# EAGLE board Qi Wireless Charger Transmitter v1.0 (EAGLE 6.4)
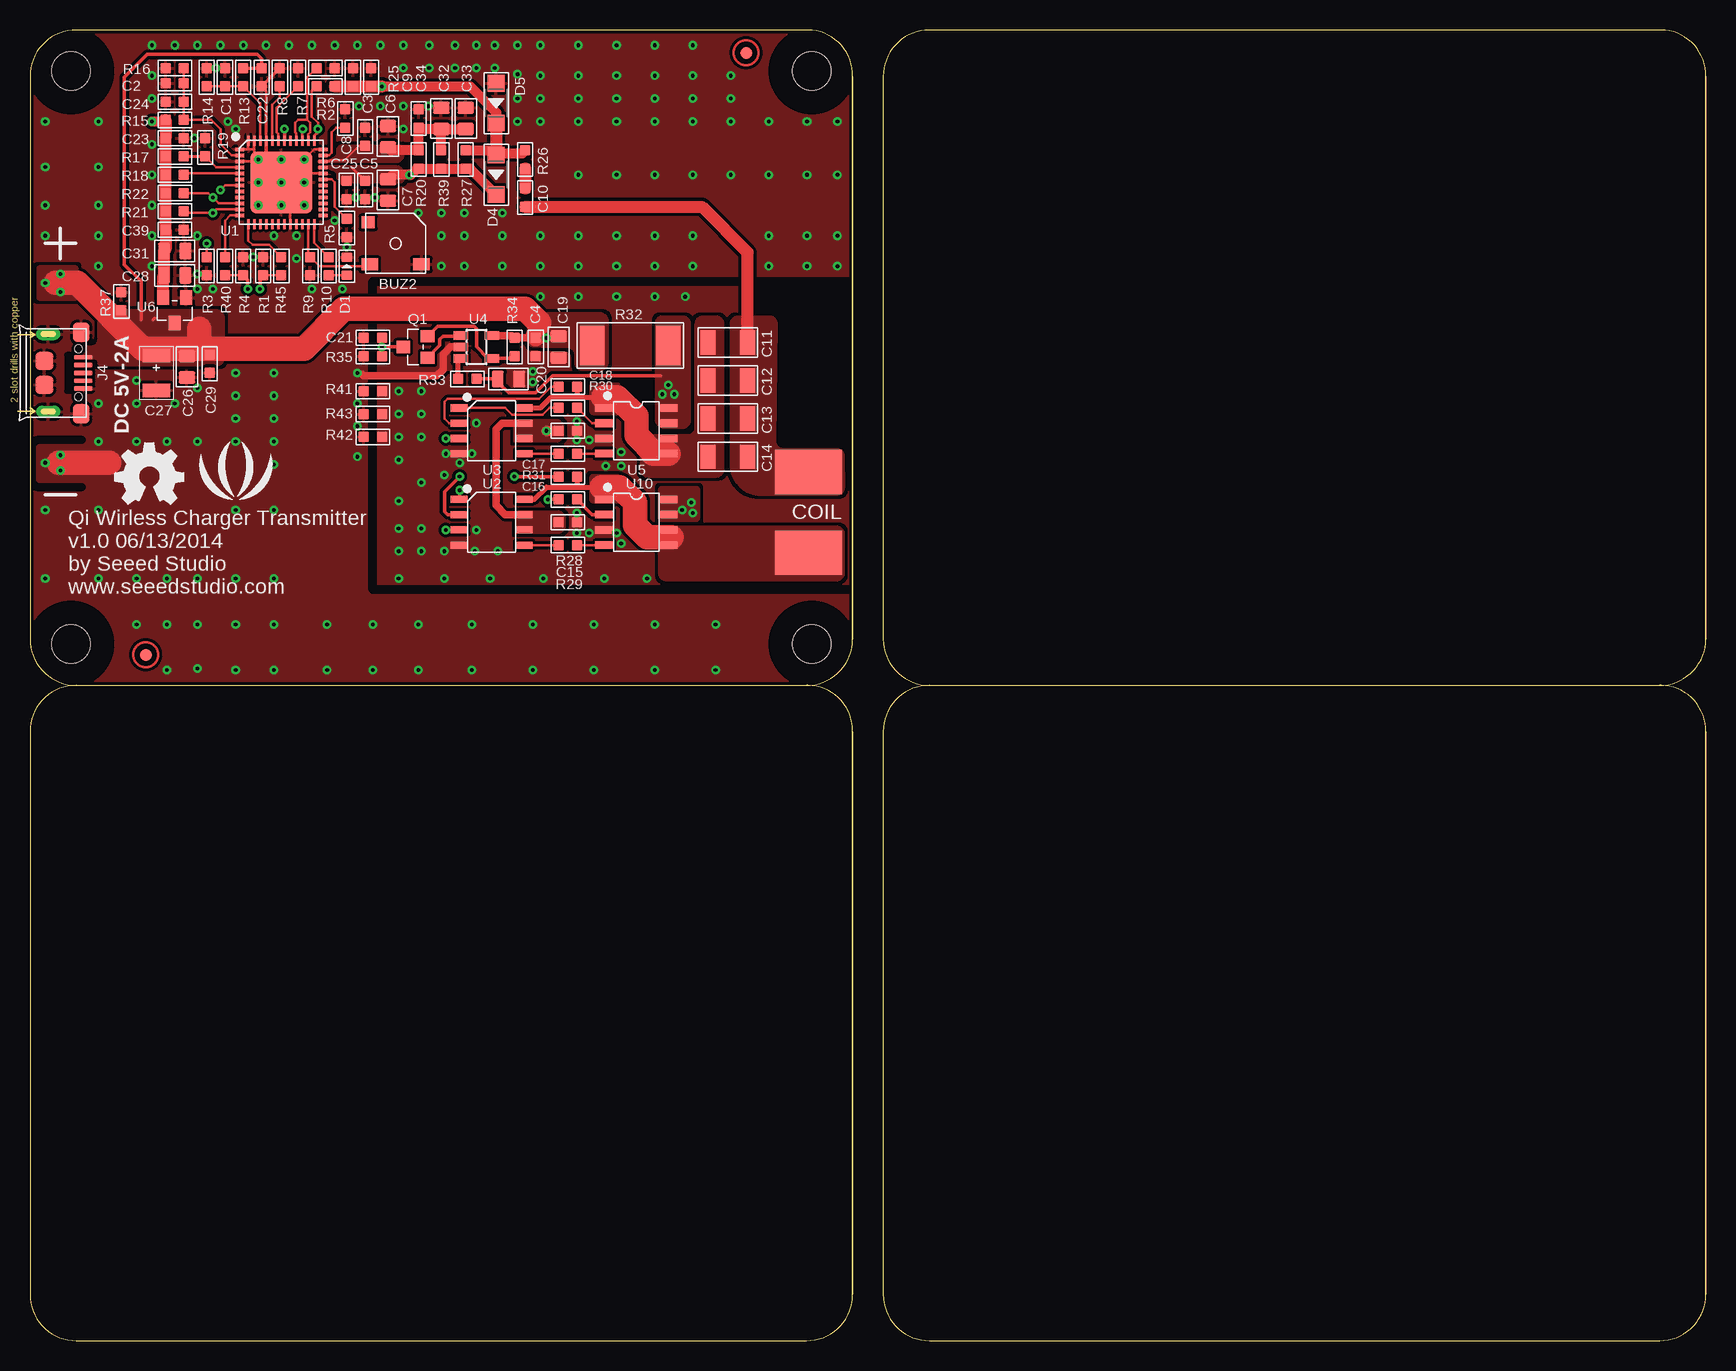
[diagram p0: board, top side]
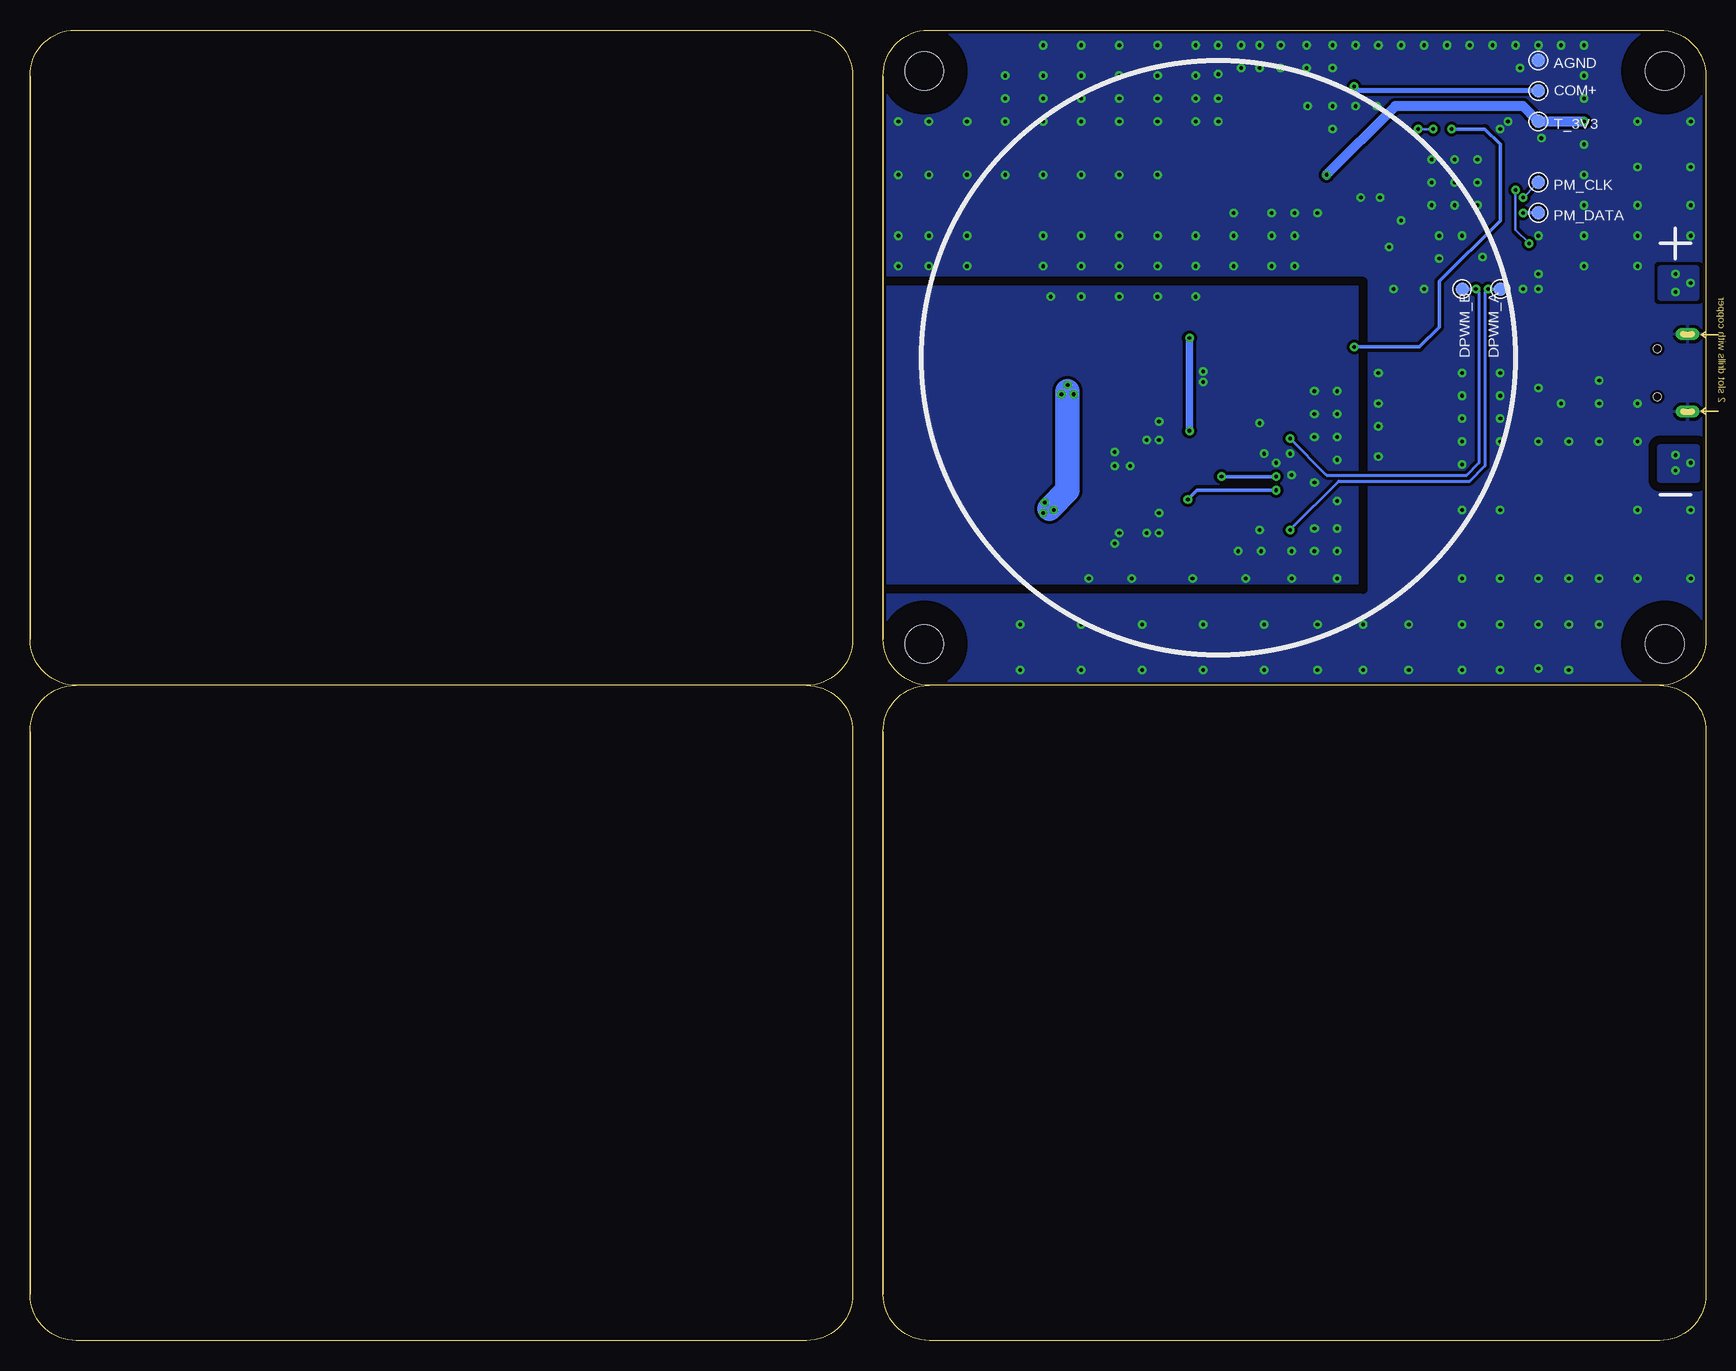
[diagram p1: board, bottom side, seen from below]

Size 139.7 x 109.22 mm. Coordinates in mm from the lower left corner, seen from the top.
Outline: 3.86,54.61 arc-90 0,58.47 0,105.36 arc-90 3.86,109.22 64.85,109.22 arc-90 68.58,105.36 68.58,58.47 arc-90 64.72,54.61
Outline: 3.86,54.61 64.72,54.61
Outline: 64.72,54.61 64.85,54.61 arc-90 68.58,50.75 68.58,3.86 arc-90 64.72,0 3.86,0 arc-90 0,3.86 0,50.75 arc-90 3.86,54.61
Outline: 68.58,50.75 68.58,3.86
Outline: 68.58,105.36 68.58,58.47
Outline: 74.98,54.61 arc-90 71.12,58.47 71.12,105.36 arc-90 74.98,109.22 135.97,109.22 arc-90 139.7,105.36 139.7,58.47 arc-90 135.84,54.61
Outline: 74.98,54.61 135.84,54.61
Outline: 135.84,54.61 135.97,54.61 arc-90 139.7,50.75 139.7,3.86 arc-90 135.84,0 74.98,0 arc-90 71.12,3.86 71.12,50.75 arc-90 74.98,54.61
Outline: 139.7,50.75 139.7,3.86
Outline: 139.7,105.36 139.7,58.47
Copper layers (1*16): Top 0.035mm / dielectric 1.5mm / Bottom 0.035mm
Design rules "default *": minimum track width 8mil, minimum drill 12mil, track to track 6mil, track to pad 6mil, pad to pad 6mil, via to via 6mil, smd to smd 0mil, copper to edge 10mil, drill to drill 8mil, minimum pad ring 10mil, minimum via ring 8mil, stop-mask expansion 4mil, vias tented up to drill 25mil, thermal gap 10mil
Net classes: 0 default: width 0.003 mm, drill 0.254 mm, clearance 0.152 mm
Holes 3.2 mm at 3.43,105.79 3.43,58.04 65.15,58.04 65.15,105.79
Holes 2.03 mm at 7.62,113.66 132.08,113.66 132.08,-4.45 7.62,-4.45
tRestrict: area 0.2,102.5 to 6.7,109; area 0.2,54.8 to 6.7,61.3; area 61.9,54.8 to 68.4,61.3; area 61.9,102.5 to 68.4,109; 9 lines
bRestrict: area 0.2,102.5 to 6.7,109; area 0.2,54.8 to 6.7,61.3; area 61.9,54.8 to 68.4,61.3; area 61.9,102.5 to 68.4,109; 12 lines

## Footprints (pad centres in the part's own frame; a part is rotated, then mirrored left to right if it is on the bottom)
TP_4545 = smd 1.143 x 1.143: T 0,0
3P-5X5X2.5H = smd 1.4 x 1: + -2.15,-1.75; - 2.15,-1.75 | smd 1.1 x 1: NC -2.3,1.75
C0603 = smd 0.889 x 0.889: 1 -0.762,0; 2 0.762,0
C0805 = smd 1.016 x 1.397: 1 -0.889,0; 2 0.889,0
C1206 = smd 1.27 x 2.032: 1 -1.651,0; 2 1.651,0
AVX-B = smd 1.143 x 2.286: + -1.46,0; - 1.46,0
1P-220X140 = smd 5.588 x 3.683: P$1 0,0
LED-0603 = smd 0.762 x 0.889: + -0.762,0; - 0.762,0
SOD123 = smd 1.397 x 1.397: + -1.651,0; - 1.651,0
MICRO-USB = smd 0.381 x 1.524: 1 -1.3,-0.25; 2 -0.65,-0.25; 3 0,-0.25; 4 0.65,-0.25; 5 1.3,-0.25 | smd 1.6 x 1.397: S1 -3.4,-0.427; S6 3.4,-0.427 | drill 0.508 pad 1.016 long: S2 -3.226,-3.175; S5 3.226,-3.175 | smd 1.5 x 1.5: S3 -1,-3.5; S4 1,-3.5 | hole 0.635: -2,-0.65; 2,-0.65
ROUND-MARK-1.0 = smd 1.016 x 1.016: P$1 0,0
SOT23 = smd 1.016 x 1.143: 1 -0.889,-1.016; 2 0.889,-1.016; 3 0,1.016
R0603 = smd 0.889 x 0.889: 1 -0.762,0; 2 0.762,0
R2512 = smd 2.032 x 3.302: 1 -3.175,0; 2 3.175,0
VQFN48 = smd 0.85 x 0.28: 1 -3.475,2.75; 2 -3.475,2.25; 3 -3.475,1.75; 4 -3.475,1.25; 5 -3.475,0.75; 6 -3.475,0.25; 7 -3.475,-0.25; 8 -3.475,-0.75; 9 -3.475,-1.25; 10 -3.475,-1.75; 11 -3.475,-2.25; 12 -3.475,-2.75; 25 3.475,-2.75; 26 3.475,-2.25; 27 3.475,-1.75; 28 3.475,-1.25; 29 3.475,-0.75; 30 3.475,-0.25; 31 3.475,0.25; 32 3.475,0.75; 33 3.475,1.25; 34 3.475,1.75; 35 3.475,2.25; 36 3.475,2.75 | smd 0.28 x 0.85: 13 -2.75,-3.475; 14 -2.25,-3.475; 15 -1.75,-3.475; 16 -1.25,-3.475; 17 -0.75,-3.475; 18 -0.25,-3.475; 19 0.25,-3.475; 20 0.75,-3.475; 21 1.25,-3.475; 22 1.75,-3.475; 23 2.25,-3.475; 24 2.75,-3.475; 37 2.75,3.475; 38 2.25,3.475; 39 1.75,3.475; 40 1.25,3.475; 41 0.75,3.475; 42 0.25,3.475; 43 -0.25,3.475; 44 -0.75,3.475; 45 -1.25,3.475; 46 -1.75,3.475; 47 -2.25,3.475; 48 -2.75,3.475 | smd 5.15 x 5.15: PAD 0,0
SOIC8-6.0 = smd 0.6 x 1.4: 1 -1.905,-2.7; 2 -0.635,-2.7; 3 0.635,-2.7; 4 1.905,-2.7; 5 1.905,2.7; 6 0.635,2.7; 7 -0.635,2.7; 8 -1.905,2.7
SOT23-5 = smd 0.69 x 1.2: 1 -0.95,-1.3; 2 0,-1.3; 3 0.95,-1.3; 4 0.95,1.3; 5 -0.95,1.3
SOP8 = smd 0.635 x 1.524: 1 -1.905,-2.667; 2 -0.635,-2.667; 3 0.635,-2.667; 4 1.905,-2.667; 5 1.905,2.667; 6 0.635,2.667; 7 -0.635,2.667; 8 -1.905,2.667
SOT23' = smd 1.016 x 1.2: 1 -0.95,-1.06; 2 0.95,-1.06; 3 0,1.06

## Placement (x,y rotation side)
AGND  DNP  [TP_4545]  13.97,106.68 0 bottom
BUZ2  KS-SMD-050025  [3P-5X5X2.5H]  30.48,91.44 0 top
C1  4.7nF  [C0603]  16.26,105.28 270 top
C2  4.7nF  [C0603]  12.06,104.78 0 top
C3  100nF  [C0603]  27.94,100.33 270 top
C4  100nF  [C0603]  42.16,82.8 270 top
C5  100nF  [C0603]  27.94,95.88 270 top
C6  4.7uF  [C0805]  29.85,100.33 270 top
C7  4.7uF  [C0805]  29.85,95.88 270 top
C8  1uF  [C0603]  26.29,101.85 90 top
C9  33pF  [C0603]  28.45,105.28 90 top
C10  4.7nF  [C0603]  41.27,95.25 270 top
C11  100nF  [C1206]  58.17,83.19 0 top
C12  100nF  [C1206]  58.17,80.01 0 top
C13  100nF  [C1206]  58.17,76.84 0 top
C14  100nF  [C1206]  58.17,73.66 0 top
C15  100nF  [C0603]  44.83,68.2 0 top
C16  100nF  [C0603]  44.83,72.01 180 top
C17  100nF  [C0603]  44.83,75.82 0 top
C18  100nF  [C0603]  44.83,79.5 180 top
C19  4.7uF  [C0805]  44.07,82.8 270 top
C20  4.7uF  [C0805]  39.88,80.14 0 top
C21  100nF  [C0603]  28.58,83.57 0 top
C22  100nF  [C0603]  19.3,105.28 90 top
C23  4.7nF  [C0603]  12.06,100.2 180 top
C24  100nF  [C0603]  12.06,103.25 0 top
C25  4.7nF  [C0603]  26.42,95.88 270 top
C26  10uF  [C0805]  13.08,81.15 90 top
C27  DNP  [AVX-B]  10.54,80.64 270 top
C28  2.2uF  [C0805]  12.06,88.77 180 top
C29  100nF  [C0603]  14.99,81.41 90 top
C31  10uF  [C0805]  12.06,90.81 180 top
C32  4.7uF  [C0805]  34.29,101.85 270 top
C33  4.7uF  [C0805]  36.32,101.85 270 top
C34  DNP  [C0603]  32.39,101.85 90 top
C39  4.7nF  [C0603]  12.06,92.58 0 top
COII2  [1P-220X140]  64.9,65.66 0 top
COIL1  [1P-220X140]  64.9,72.39 0 top
COM+  DNP  [TP_4545]  13.97,104.14 0 bottom
D1  RED  [LED-0603]  26.42,89.53 90 top
D4  MBR0520LT1G  [SOD123]  38.86,97.16 270 top
D5  MBR0520LT1G  [SOD123]  38.86,103.12 270 top
DPWM_A  DNP  [TP_4545]  17.15,87.63 0 bottom
DPWM_B  DNP  [TP_4545]  20.32,87.63 0 bottom
J4  MICRO-B-SMD_340005001  [MICRO-USB]  4.7,80.64 270 top
P1  [ROUND-MARK-1.0]  9.65,57.15 0 top
P2  [ROUND-MARK-1.0]  59.69,107.31 0 top
P3  [ROUND-MARK-1.0]  not placed on the board
P4  [ROUND-MARK-1.0]  not placed on the board
P5  [ROUND-MARK-1.0]  not placed on the board
P6  [ROUND-MARK-1.0]  not placed on the board
PM_CLK  DNP  [TP_4545]  13.97,96.52 0 bottom
PM_DATA  DNP  [TP_4545]  13.97,93.98 0 bottom
Q1  MMBT3906LT3G  [SOT23]  32.13,82.8 90 top
R1  10K  [R0603]  19.43,89.53 90 top
R2  10R  [R0603]  24.64,104.52 180 top
R3  DNP  [R0603]  14.73,89.53 270 top
R4  10K  [R0603]  17.78,89.53 90 top
R5  DNP  [R0603]  26.42,92.71 270 top
R6  10R  [R0603]  24.64,106.05 180 top
R7  DNP  [R0603]  22.35,105.28 90 top
R8  42.2K  [R0603]  20.83,105.28 90 top
R9  10K  [R0603]  23.37,89.53 270 top
R10  470R  [R0603]  24.89,89.53 270 top
R13  75K  [R0603]  17.78,105.28 270 top
R14  10K  [R0603]  14.73,105.28 270 top
R15  100K  [R0603]  12.06,101.73 180 top
R16  DNP  [R0603]  12.06,106.05 0 top
R17  100K  [R0603]  12.06,98.68 180 top
R18  10K  [R0603]  12.06,97.16 180 top
R19  DNP  [R0603]  14.61,99.44 90 top
R20  DNP  [R0603]  32.39,98.42 270 top
R21  10K  [R0603]  12.06,94.11 180 top
R22  10K  [R0603]  12.06,95.63 180 top
R25  10K  [R0603]  26.92,105.28 90 top
R26  100K  [R0603]  41.27,98.42 270 top
R27  22K  [R0603]  36.32,98.42 270 top
R28  10R  [R0603]  44.83,70.1 180 top
R29  0R  [R0603]  44.83,66.29 180 top
R30  10R  [R0603]  44.83,77.72 180 top
R31  0R  [R0603]  44.83,73.91 180 top
R32  20mR_1%  [R2512]  50.04,82.93 0 top
R33  200R  [R0603]  36.45,80.14 180 top
R34  200R  [R0603]  40.39,82.8 270 top
R35  10K  [R0603]  28.58,82.04 0 top
R37  1M  [R0603]  7.62,86.61 270 top
R39  10R  [R0603]  34.29,98.42 270 top
R40  10R  [R0603]  16.26,89.53 270 top
R41  0R  [R0603]  28.58,79.12 180 top
R42  0R  [R0603]  28.58,75.31 180 top
R43  0R  [R0603]  28.58,77.22 180 top
R45  10R  [R0603]  20.96,89.53 270 top
T_3V3  DNP  [TP_4545]  13.97,101.6 0 bottom
U1  BQ500211RGZ  [VQFN48]  20.96,96.52 0 top
U2  TPS28225  [SOIC8-6.0]  38.48,68.2 270 top
U3  TPS28225  [SOIC8-6.0]  38.48,75.82 270 top
U4  OPA333DBV  [SOT23-5]  37.21,82.8 270 top
U5  CJQ9926  [SOP8]  50.55,75.82 270 top
U6  XC6206MR  [SOT23']  12.06,85.85 180 top
U10  CJQ9926  [SOP8]  50.55,68.2 270 top
U$10  [OSHW_FILLX200_NOTEXT]  7.11,69.72 0 top
U$15  [LOGO_SILK]  17.15,71.75 0 top

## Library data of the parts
AGND COM+ DPWM_A DPWM_B P1-P6 PM_CLK PM_DATA T_3V3 = Discrete; PARTNO: DNP
BUZ2 U1-U3 = template
C1-C29 C31-C34 C39 COII2 COIL1 D1 Q1 R1-R10 R13-R22 R25-R35 R37 R39-R43 R45 U5 U10 = Discrete
D4 D5 = OPL
J4 = Connector 
U4 U6 = IC
U$10 U$15 = Logo

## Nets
3V3_ADC: C3.2 C6.2 C32.2 C33.2 C34.1 R20.1 R39.1 U1.34
3V3_VCC: C5.1 C7.1 C23.2 C25.1 C28.2 C31.2 C39.1 D4.- R15.2 R17.2 R18.2 R20.2 R21.2 R22.2 R27.2 R39.2 T_3V3.T U1.33 U6.2
AGND: AGND.T BUZ2.- C1.1 C2.1 C3.1 C5.2 C6.1 C7.2 C8.2 C9.2 C21.1 C22.1 C23.1 C24.1 C25.2 C26.1 C27.- C28.1 C29.1 C31.1 C32.1 C33.1 C34.2 C39.2 D1.- D5.+ J4.5 J4.S1 J4.S2 J4.S3 J4.S4 J4.S5 J4.S6 R1.2 R3.2 R4.2 R5.2 R6.1 R7.2 R8.2 R9.2 R14.1 R16.1 R19.2 R25.2 R35.1 R37.1 R41.2 R42.2 R43.2 U1.1 U1.3 U1.20 U1.32 U1.36 U1.45 U1.47 U1.48 U1.PAD U4.2 U6.1
COMM+: R2.2 U1.37 U1.39
COMM-: R6.2 U1.38 U1.40
DPWM_1A: DPWM_A.T R4.1 R40.2 U2.3
DPWM_1B: DPWM_B.T R1.1 R45.2 U3.3
GND: C4.2 C15.2 C17.2 C19.2 C20.2 R41.1 R42.1 R43.1 U2.4 U3.4 U5.3 U10.3
I_SENSE: C21.2 Q1.3 R35.2 U1.42
LOSS_THR: R7.1 U1.43
MCU_MOSI: U1.25
MCU_RDY: U1.26
MCU_SYNC: U1.14
N$2: R5.1 U1.31
N$3: R3.1 U1.7
N$5: R45.1 U1.13
N$6: R40.1 U1.12
N$7: C9.1 COM+.T D4.+ D5.- R2.1 R25.1 R26.1 R27.1
N$8: R33.2 U4.3
N$10: C2.2 C24.2 R15.1 R16.2 U1.2
N$11: C10.1 R26.2
N$12: R8.1 U1.44
N$13: BUZ2.+ R9.1 U1.23
N$14: D1.+ R10.2
N$15: R10.1 U1.24
N$17: C8.1 U1.35
N$18: R29.2 U2.5
N$19: R18.1 U1.5
N$20: R17.1 R19.1 U1.4
N$21: R28.2 U2.1
N$22: C18.2 U3.2
N$24: C16.1 COII2.P$1 U2.8 U10.1 U10.5 U10.6
N$25: R28.1 U10.2
N$27: Q1.2 R34.2 U4.4
N$28: R29.1 U10.4
N$29: C16.2 U2.2
N$30: R31.2 U3.5
N$31: R30.1 U5.2
N$33: R31.1 U5.4
N$34: R30.2 U3.1
N$35: C11.1 C12.1 C13.1 C14.1 C18.1 U3.8 U5.1 U5.5 U5.6
N$37: C10.2 C11.2 C12.2 C13.2 C14.2 COIL1.P$1
N$40: C20.1 R32.2 R33.1 U5.7 U5.8 U10.7 U10.8
N$41: Q1.1 U4.1
PM_CLK: PM_CLK.T R22.1 U1.10
PM_DATA: PM_DATA.T R21.1 U1.11
SLEEP: U1.6
V_SENSE: C1.2 R13.2 R14.2 U1.46
VIN: C4.1 C15.1 C17.1 C19.1 C22.2 C26.2 C27.+ C29.2 J4.1 R13.1 R32.1 R34.1 R37.2 U2.6 U2.7 U3.6 U3.7 U4.5 U6.3

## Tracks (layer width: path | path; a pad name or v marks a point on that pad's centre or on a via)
3V3_ADC
  Top 0.203: C3.2 27.43,99.57 26.23,98.36 25.02,98.36 24.93,98.27 U1.34
  Top 0.813: R39.1 C32.2 | C32.2 32.51,100.97 C34.1 R20.1 30.1,99.19 C6.2 | C32.2 C33.2
  pour Top (isolate 0.203, rank 2, no thermals): 24.07,98.49 25.15,98.49 arc90 25.65,99 25.65,99.31 arc-90 26.42,99.57 30.61,99.57 arc-90 31.12,99.31 31.12,98.87 arc-90 30.48,98.23 24.07,98.23
3V3_VCC  (via drill 0.3 pad 0.64)
  Top 0.254: 26.82,97.77 C5.1
  Top 0.813: R27.2 R39.2 R20.2 32.26,97.66 31.75,97.16 v31.62,97.16 30.23,97.16 C7.1 | R27.2 36.45,97.66 | R27.2 36.7,97.66 D4.- | v10.16,101.6 11.18,101.6 R15.2
  Top 1.016: U6.2 11.11,88.71 C28.2 C31.2 11.3,90.93 C39.1 R21.2 R22.2 R18.2 R17.2 C23.2 R15.2
  Bottom 0.813: v31.62,97.16 25.91,102.87 15.24,102.87 14.61,102.23 14.6,102.23 T_3V3.T v10.16,101.6
  pour Top (isolate 0.203, rank 3, no thermals): 24.07,97.85 30.48,97.85 arc-90 31.12,97.22 31.12,96.9 arc-90 30.86,96.52 26.67,96.52 arc-90 25.65,96.65 25.65,97.09 arc90 25.15,97.6 24.07,97.6
AGND  (via drill 0.3 pad 0.64)
  Top 0.203: U1.47 18.7,98.9 19.3,98.3 | U1.1 18.62,99.27 18.67,99.31 | U1.48 18.2,99.33 18.22,99.31 | U1.3 19.02,98.27 19.05,98.3 | U1.36 23.7,99.27 21.7,97.27 | 21.7,97.27 U1.PAD 21.7,95.77 U1.20 | U1.32 21.7,97.27 | U1.45 19.7,104.12 C22.1
  Top 0.305: U1.45 19.7,98.44 19.68,98.42 | R8.2 C22.1
  Top 0.61: U4.2 35.05,82.8 34.42,82.17 34.42,80.9 33.91,80.39 27.81,80.39 27.69,80.52 | v1.27,73.15 2.41,73.15
  Top 2.032: 2.41,73.15 6.6,73.15
  other vias: 10.16,103.5 10.16,105.41 10.16,94.62 13.97,92.08 15.49,106.05 13.97,107.95 15.88,107.95 21.59,107.95 23.5,107.95 25.4,107.95 27.31,107.95 29.21,107.95 31.12,107.95 33.27,107.95 35.43,107.95 37.21,107.95 38.73,107.95 40.64,107.95 31.12,106.05 33.27,106.05 35.43,106.05 37.21,106.05 38.73,106.05 40.64,105.54 40.64,103.5 42.55,107.95 42.55,105.41 42.55,103.5 42.55,101.6 32.39,93.98 26.42,91.12 36.2,93.98 36.2,92.08 34.29,93.98 39.37,92.08 39.37,93.98 42.55,92.08 15.24,87.63 10.16,89.53 10.16,92.08 8.89,78.11 20.32,80.64 22.23,90.17 18.61,90.3 22.23,92.08 20.32,92.08 10.16,107.95 12.06,107.95 29.21,102.87 27.43,102.87 31.12,102.87 31.12,100.97 40.64,101.6 20.32,69.22 20.32,63.5 20.32,73.03 20.32,74.93 20.32,76.84 20.32,78.74 1.27,69.22 5.71,69.22 17.15,69.22 17.15,63.5 17.15,59.69 20.32,59.69 17.15,74.93 17.15,76.84 17.15,78.74 17.15,80.64 5.71,97.79 5.71,94.62 5.71,92.08 5.71,89.53 1.27,92.08 1.27,94.62 1.27,97.79 5.71,101.6 1.27,101.6 5.71,74.93 5.71,78.11 8.89,80.01 12.06,78.11 13.97,79.38 8.89,74.93 11.43,74.93 13.97,74.93 1.27,63.5 5.71,63.5 11.43,63.5 8.89,63.5 13.97,63.5 17.15,55.88 20.32,55.88 39.37,89.53 42.55,89.53 45.72,92.08 48.9,92.08 55.25,92.08 48.9,89.53 45.72,89.53 52.07,89.53 55.25,89.53 45.72,97.16 48.9,97.16 55.25,97.16 52.07,97.16 55.25,101.6 52.07,101.6 48.9,101.6 45.72,101.6 45.72,103.5 52.07,107.95 45.72,105.41 45.72,107.95 13.97,59.69 8.89,59.69 13.97,56.01 11.43,59.69 11.43,55.88 24.77,59.69 26.04,87.63 23.5,87.63 28.58,59.69 32.39,59.69 36.83,59.69 41.91,59.69 46.99,59.69 13.72,100.2 10.16,99.69 20.96,96.52 22.86,98.42 19.05,98.42 19.05,94.62 22.86,94.62 20.96,98.42 20.96,94.62 22.86,96.52 19.05,96.52 24.77,55.88 28.58,55.88 32.39,55.88 36.83,55.88 41.91,55.88 46.99,55.88 52.07,92.08 55.25,107.95 58.42,101.6 61.59,101.6 64.77,101.6 67.31,101.6 58.42,97.16 61.59,97.16 64.77,97.16 67.31,97.16 61.59,92.08 64.77,92.08 67.31,92.08 61.59,89.53 64.77,89.53 67.31,89.53 48.9,107.95 48.9,105.41 52.07,105.41 55.25,105.41 55.25,103.5 52.07,103.5 48.9,103.5 2.54,73.79 2.54,72.52 52.07,59.69 52.07,55.88 57.15,59.69 57.15,55.88 58.42,103.5 58.42,105.41 10.16,97.16 13.97,87.63 17.78,107.95 19.69,107.95 36.2,89.53 34.29,89.53 34.29,92.08 27.31,80.64 27.31,78.11 27.31,76.2 33.21,102.87 27.31,73.66 28.77,95.25 27.18,95.25 13.97,88.9 25.4,93.34 16.51,101.6 17.15,100.97
  pour Top (isolate 0.254, rank 6): 0,54.61 69.21,54.61 69.21,109.22 0,109.22
  pour Bottom (isolate 0.254, rank 6): 0,54.61 69.21,54.61 69.21,109.22 0,109.22
  pour Bottom (isolate 0.254, no thermals): 4.19,73.91 4.19,72.39 arc-90 3.43,71.75 1.27,71.75 arc-90 0.89,72.39 0.89,73.91 arc-90 1.27,74.55 3.43,74.55 arc-90
COMM+  (via drill 0.3 pad 0.64)
  Top 0.203: R2.2 23.49,104.14 23.49,101.98 24,101.47 v24,100.97 24,100.71 23.7,100.41 U1.37 | U1.39 22.7,100.94 v22.73,100.97
  Bottom 0.203: v22.73,100.97 v24,100.97
COMM-
  Top 0.203: U1.38 23.2,100.55 23.37,100.71 23.37,101.47 23.11,101.73 | 23.11,101.73 23.11,105.28 R6.2 | U1.40 22.2,100.6 22.1,100.71 22.1,101.47 22.35,101.73 22.86,101.73 22.99,101.73 | 22.99,101.73 23.11,101.73 | 22.99,101.73 23.11,101.85
DPWM_1A  (via drill 0.3 pad 0.64)
  Top 0.203: R4.1 R40.2
  Top 0.254: v34.67,67.56 U2.3
  Top 0.305: v18.16,87.63 18.16,88.39 R4.1
  Bottom 0.254: v34.67,67.56 30.61,71.63 19.68,71.63 18.41,72.9 18.41,87.38 v18.16,87.63
  Bottom 0.305: DPWM_A.T v18.16,87.63
DPWM_1B  (via drill 0.3 pad 0.64)
  Top 0.203: R1.1 R45.2
  Top 0.305: U3.3 v34.67,75.18 | v19.18,87.63 19.18,88.52 R1.1
  Bottom 0.254: v34.67,75.18 31.62,72.14 19.94,72.14 18.92,73.15 18.92,87.38 v19.18,87.63
  Bottom 0.305: DPWM_B.T v19.18,87.63
GND  (via drill 0.3 pad 0.64)
  other vias: 34.67,73.91 32.64,77.22 35.81,73.15 37.21,76.45 36.83,73.91 32.64,65.79 34.54,65.79 37.08,65.79 37.21,67.56 45.59,67.31 46.61,67.31 45.59,68.96 49.28,66.42 48.9,67.31 46.61,75.06 45.59,75.06 45.59,76.58 38.99,65.79 45.72,87 48.9,87 52.07,87 54.61,87 30.73,63.5 34.54,63.5 38.35,63.5 42.8,63.5 47.88,63.5 32.64,67.69 30.73,67.69 30.73,69.98 32.64,71.5 34.54,72.14 32.64,75.31 30.73,73.41 30.73,75.31 30.73,77.22 30.73,79.12 32.64,79.12 30.73,65.79 49.28,74.04 48.01,72.9 49.28,72.9 41.91,79.88 41.91,80.77 51.44,63.5 42.55,87
  pour Bottom (isolate 0.254, rank 5, no thermals): 28.58,88.27 68.58,88.27 68.58,62.87 28.58,62.87
  pour Top (isolate 0.254, rank 5, no thermals): 28.58,88.27 68.58,88.27 68.58,62.87 28.58,62.87
I_SENSE  (via drill 0.3 pad 0.64)
  Top 0.305: v21.21,100.97 U1.42 | C21.2 v29.34,82.8 | v29.34,82.8 R35.2 | v29.34,82.8 Q1.3
  Bottom 0.305: v29.34,82.8 23.88,82.8 22.23,84.45 22.23,88.27 17.15,93.34 17.15,99.69 18.42,100.97 v21.21,100.97
LOSS_THR
  Top 0.203: U1.43 20.7,100.58 20.57,100.71 20.57,102.74 R7.1
N$2
  Top 0.203: U1.31 25.15,96.77 25.4,96.52 25.4,94.49 R5.1
N$3  (via drill 0.3 pad 0.64)
  Top 0.203: U1.7 16.26,96.27 v15.87,95.88 | v14.73,91.44 R3.1
  Bottom 0.203: v15.87,95.88 15.87,92.58 v14.73,91.44
N$5
  Top 0.203: U1.13 18.2,91.65 18.54,91.31 19.94,91.31 R45.1
N$6
  Top 0.203: U1.12 16.7,93.77 16.26,93.33 R40.1
N$7  (via drill 0.3 pad 0.64)
  Top 0.813: R27.1 38.86,99.19 38.99,99.06 38.99,98.93 | 38.99,98.93 41.02,98.93 R26.1 | 38.99,98.93 D4.+ | v29.34,104.52 36.7,104.52 38.86,102.36 38.86,101.09
  Top 1.016: R2.1 R25.1 C9.1 v29.34,104.52 | D4.+ 38.86,101.09 D5.-
  Bottom 0.406: COM+.T 28.96,104.14 v29.34,104.52
N$8
  Top 0.406: R33.2 35.69,81.63 U4.3
N$10
  Top 0.203: R16.2 C2.2 C24.2 R15.1 15.11,101.73 15.87,100.97 15.87,99.69 16.8,98.77 U1.2
N$11
  Top 1.016: R26.2 C10.1
N$12
  Top 0.203: U1.44 20.2,103.01 20.83,103.63 R8.1
N$13
  Top 0.203: BUZ2.+ 28.17,89.53 24.13,89.53 R9.1 23.2,90.46 U1.23
N$14
  Top 0.203: R10.2 D1.+
N$15
  Top 0.203: U1.24 23.7,91.48 R10.1
N$17
  Top 0.203: U1.35 24.94,98.77 25.15,98.98 25.15,100.71 25.53,101.09 C8.1
N$18
  Top 0.203: U2.5 R29.2
N$19
  Top 0.203: U1.5 12.94,97.27 R18.1
N$20
  Top 0.203: U1.4 15.51,97.77 R19.1
  Top 0.254: R17.1 R19.1
N$21  (via drill 0.3 pad 0.64)
  Top 0.305: R28.2 v43.18,70.1 | v35.81,70.87 35.81,70.14 U2.1
  Bottom 0.305: v35.81,70.87 42.42,70.87 v43.18,70.1
N$22
  Top 0.203: U3.2 34.92,76.45 34.54,76.84 34.54,78.23 34.8,78.49 42.42,78.49 43.43,79.5 C18.2 44.2,79.5
N$24
  Top 0.406: U2.8 42.04,70.1 43.05,71.12 45.47,71.12 | 45.47,71.12 45.72,71.12 | C16.1 45.59,71.25 | 45.59,71.25 45.47,71.12 | 45.59,71.25 45.72,71.12 | U10.1 47.88,70.99 | 45.72,71.12 47.62,71.12 47.88,71.12 47.88,70.87
  Top 2.032: 47.62,71.12 49.15,71.12 50.42,69.85 50.42,67.95 51.44,66.93 53.47,66.93
  pour Top (isolate 0.254, no thermals): 67.18,63.37 53.09,63.37 arc-90 52.45,64.01 52.45,67.18 arc-90 53.09,67.82 67.18,67.82 arc-90 67.82,67.18 67.82,64.01 arc-90
  pour Top (isolate 0.254, no thermals): 46.74,71.88 46.74,70.1 arc90 46.99,69.85 49.15,69.85 49.15,71.88 arc90 48.9,72.14 46.99,72.14 arc90
N$25
  Top 0.305: U10.2 46.86,68.83 R28.1
N$27
  Top 0.305: 40.51,82.17 R34.2 40.2,81.85 U4.4 38.16,81.85 37.21,82.8 37.21,84.33 37.02,84.52 33.97,84.52 Q1.2
N$28
  Top 0.203: R29.1 U10.4
N$29  (via drill 0.3 pad 0.64)
  Top 0.305: U2.2 34.8,68.83 34.54,69.09 34.54,70.74 v35.81,72.01 | v40.39,72.01 C16.2
  Bottom 0.305: v35.81,72.01 v40.39,72.01
N$30
  Top 0.203: U3.5 R31.2
N$31
  Top 0.203: U5.2 46.86,76.45 R30.1
N$33
  Top 0.203: R31.1 U5.4
N$34
  Top 0.203: U3.1 39.62,77.72 40.2,77.15 42.74,77.15 43.31,77.72 R30.2
N$35
  Top 0.406: U3.8 42.54,77.72 43.43,78.61 45.59,78.61 | C18.1 45.59,78.61 | 45.59,78.61 47.75,78.61 47.88,78.61 U5.1
  Top 2.032: 47.75,78.61 48.95,78.61 50.55,77.01 50.55,75.44 52.07,73.91 | U5.5 52.07,73.91 | 52.07,73.91 51.94,73.91
  pour Top (isolate 0.254, no thermals): 50.93,72.64 50.93,74.8 arc-90 51.56,75.44 54.86,75.44 arc90 55.5,76.07 55.5,84.71 arc-90 56.13,85.34 57.15,85.34 arc-90 57.79,84.71 57.79,72.64 arc-90 57.15,72.01 51.56,72.01 arc-90
  pour Top (isolate 0.254, no thermals): 46.74,79.5 46.74,77.47 arc90 46.99,77.22 48.9,77.22 arc90 49.15,77.47 49.15,79.5 arc90 48.9,79.76 46.99,79.76 arc90
N$37
  Top 1.016: C11.2 59.82,90.68 56.01,94.49 C10.2
  pour Top (isolate 0.254, no thermals): 67.2,70.49 60.96,70.49 arc-90 58.42,73.03 58.42,84.71 arc-90 59.05,85.34 61.59,85.34 arc-90 62.23,84.71 62.1,74.93 arc90 62.74,74.3 67.19,74.3 arc-90 67.82,73.66 67.84,71.13 arc-90
N$40  (via drill 0.3 pad 0.64)
  Top 0.305: 52.96,82.68 R32.2 | 52.58,80.39 43.56,80.39 42.16,78.99 39.88,78.99 38.99,79.88 C20.1 R33.1
  Bottom 0.203: 53.21,79.12 52.96,79.12 v52.7,78.87
  Bottom 0.61: 54.74,69.34 54.48,69.34 v54.36,69.22
  Bottom 2.032: 53.21,79.12 53.21,70.87 54.74,69.34
  other vias: 53.21,79.63 53.72,78.87 55.25,68.96 55.12,69.85
  pour Top (isolate 0.254, no thermals): 52.2,76.71 52.2,84.71 arc-90 52.7,85.34 54.36,85.34 arc-90 54.99,84.71 54.99,76.71 arc-90 54.36,76.07 52.96,76.07 arc-90
  pour Top (isolate 0.254, no thermals): 55.5,68.33 52.7,68.33 arc-90 52.45,68.58 52.45,70.87 arc-90 52.7,71.12 55.5,71.12 arc-90 55.75,70.87 55.75,68.58 arc-90
N$41
  Top 0.305: U4.1 35.85,83.69 34.42,83.69 34.16,83.44 34.16,82.93 Q1.1
PM_CLK  (via drill 0.3 pad 0.64)
  Top 0.203: U1.10 15.72,94.77 v15.24,95.25 14.86,95.63 R22.1
  Bottom 0.203: PM_CLK.T 13.97,96.27 14.22,96.27 v15.24,95.25
PM_DATA  (via drill 0.3 pad 0.64)
  Top 0.203: U1.11 15.53,94.27 v15.24,93.98 12.95,93.98 R21.1
  Bottom 0.305: PM_DATA.T v15.24,93.98
V_SENSE
  Top 0.203: U1.46 19.2,103.1 R13.2 C1.2 R14.2
VIN  (via drill 0.3 pad 0.64)
  Top 0.305: 7.87,85.47 7.75,85.34 | 10.41,85.22 10.29,85.09 | 9.27,85.09 9.27,88.27 7.87,89.66 7.87,105.28 9.78,107.19 18.92,107.19 19.3,106.81 C22.2 R13.1
  Top 0.406: 7.56,85.66 7.62,85.72
  Top 0.61: U4.5 40.2,83.75 R34.1 C4.1 v43.05,83.57 | U2.7 39.62,68.83 38.86,69.6 38.86,75.95 39.37,76.45 U3.7
  Top 0.813: v43.05,75.82 C17.1
  Top 1.27: 42.42,84.84 42.42,84.2 42.04,83.82
  Top 1.422: 42.04,83.82 42.04,83.69 C4.1
  Top 2.032: 14.1,84.33 14.1,83.19 | 14.73,82.68 22.86,82.68 26.16,85.98 41.28,85.98 42.42,84.84 | 14.73,82.68 14.22,83.19 | 14.73,82.68 9.4,82.68 3.94,88.14 2.16,88.14
  Bottom 0.61: v43.05,83.57 v43.05,75.82
  other vias: 1.27,88.14 2.54,88.9 2.54,87.38
  pour Top (isolate 0.254, no thermals): 41.53,85.6 47.5,85.6 arc-90 48.13,84.96 48.13,81.53 arc-90 47.5,80.9 46.1,80.9 arc-90 45.47,81.53 45.47,82.17 arc90 44.83,82.8 42.16,82.8 arc-90 41.53,83.44
  pour Top (isolate 0.254, no thermals): 40.39,74.93 43.82,74.93 arc90 44.45,75.56 44.45,76.07 arc90 43.82,76.71 40.39,76.71
  pour Top (isolate 0.254, no thermals): 40.51,67.31 43.94,67.31 arc90 44.58,67.94 44.58,68.45 arc90 43.94,69.09 40.51,69.09
  pour Top (isolate 0.254, no thermals): 3.68,82.8 5.08,82.8 arc90 5.71,83.44 5.71,83.82 9.53,83.82 9.53,81.28 5.97,81.28 arc-90 5.71,81.53 5.71,81.6 arc90 5.46,81.85 3.68,81.85
  pour Top (isolate 0.254, no thermals): 16.13,85.22 16.13,81.91 arc-90 15.49,81.28 6.35,81.28 arc-90 5.71,81.91 5.71,85.22 arc-90 6.35,85.85 15.49,85.85 arc-90
  pour Top (isolate 0.254, no thermals): 3.68,86.74 0.89,86.74 arc-90 0.64,87 0.64,89.28 arc-90 0.89,89.53 3.68,89.53 arc-90 3.94,89.28 3.94,87 arc-90
  pour Bottom (isolate 0.254, no thermals): 3.68,86.74 0.89,86.74 arc-90 0.64,87 0.64,89.28 arc-90 0.89,89.53 3.68,89.53 arc-90 3.94,89.28 3.94,87 arc-90

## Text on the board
tPlace: DC 5V-2A | COIL | Qi Wirless Charger Transmitter | v1.0 06/13/2014 | by Seeed Studio | www.seeedstudio.com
